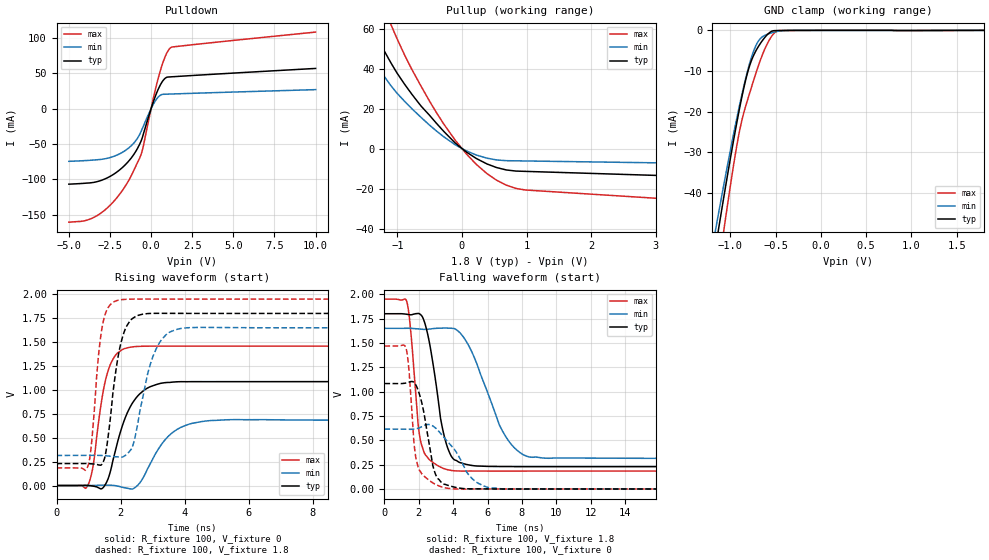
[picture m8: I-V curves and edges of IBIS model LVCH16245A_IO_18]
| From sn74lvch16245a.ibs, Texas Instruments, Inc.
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[Model]   LVCH16245A_IO_18
Model_type  3-state
Enable   Active-Low
Vref =   0
Rref =   1000
Cref =   30p
Vmeas =   0.9
| variable   typ   min   max
C_comp   4.79pF   4.43pF   5.43pF
| C_pullup   5.86pF   3.31pF   12.01pF
| C_pulldown   8.06pF   4.99pF   10.39pF
| C_tri-state   4.79pF   4.43pF   5.43pF
[Temperature Range]   40   100   -40
| Ambient temperature   25   85   -40
[Voltage range]   1.8   1.65   1.95
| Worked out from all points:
|   slope of the pulldown table from 0 to 0.27 V, typ, clamps not added: 14.8 ohm
|   slope of the pullup table from 0 to 0.27 V, typ, clamps not added: 46.5 ohm
|   GND clamp passes 1 mA (typ) near -0.59 V on its own axis
|   rising waveform, R_fixture 100, V_fixture 0: 20-80 % time 652ps typ, 803ps min, 400ps max; typ from 0 V to 1.09 V
|   falling waveform, R_fixture 100, V_fixture 1.8: 20-80 % time 843ps typ, 1.76ns min, 514ps max; typ from 1.8 V to 0.23 V
|   rising waveform, R_fixture 100, V_fixture 1.8: 20-80 % time 385ps typ, 552ps min, 277ps max; typ from 0.229 V to 1.8 V
|   falling waveform, R_fixture 100, V_fixture 0: 20-80 % time 654ps typ, 1.37ns min, 414ps max; typ from 1.08 V to 0 V
[GND Clamp]
| LVCH16245A_IO_18
|   Voltage   I(typ)   I(min)   I(max)
-5V       -657.7mA   -597mA     -758.5mA
-1.165V   -53.4mA    -49.05mA   -63.64mA
-1.13V    -48.59mA   -44.75mA   -58.04mA
-1.065V   -39.83mA   -36.93mA   -47.84mA
-915mV    -20.95mA   -20.02mA   -26.51mA
-860mV    -14.93mA   -14.46mA   -20.87mA
-795mV    -9.18mA    -8.674mA   -15.93mA
-740mV    -5.956mA   -4.853mA   -12.01mA
-675mV    -3.409mA   -2.158mA   -7.673mA
-575mV    -688.2uA   -820.5uA   -2.53mA
-495mV    -55.43uA   -321.6uA   -307.2uA
1.8V      10.89pA    55.22nA    -431pA
[Pulldown]
| LVCH16245A_IO_18
|   Voltage   I(typ)   I(min)   I(max)
-5V       -106.8mA   -74.48mA   -160.5mA
-3.945V   -105.3mA   -73.35mA   -157.9mA
-3.11V    -102mA     -71.9mA    -148.6mA
-2.215V   -91.79mA   -66.95mA   -129.7mA
-1.4V     -75.15mA   -56.3mA    -103.1mA
-920mV    -59.95mA   -44.93mA   -80.72mA
-585mV    -44.32mA   -30.88mA   -63.04mA
60mV      4.341mA    2.845mA    6.529mA
455mV     28.54mA    16.86mA    44.89mA
845mV     42.74mA    20.36mA    72.96mA
1.185V    44.91mA    20.64mA    86.07mA
10V       56.83mA    26.86mA    108.2mA
[Pullup]
| LVCH16245A_IO_18
|   Voltage   I(typ)   I(min)   I(max)
-5V       59.9mA     24.93mA    137.1mA
-3.525V   172.8mA    34.3mA     282.6mA
-3.275V   178.8mA    43.79mA    262.1mA
-3.19V    174.9mA    62.85mA    254.7mA
-1.815V   89.03mA    67.09mA    127mA
-1.63V    76.68mA    57.69mA    108.5mA
-1.365V   58.9mA     44.05mA    84.12mA
-1.1V     43.06mA    31.59mA    62.31mA
-105mV    2.886mA    1.98mA     4.306mA
390mV     -7.662mA   -4.752mA   -12.55mA
835mV     -11.19mA   -6.053mA   -19.89mA
10V       -20.36mA   -10.29mA   -39.14mA
[Ramp]
| LVCH16245A_IO_18
| variable   typ   min   max
dV/dt_r   0.67/6.76E-10   0.44/8.65E-10   0.89/4.15E-10
dV/dt_f   0.94/9.08E-10   0.80/1.91E-09   1.06/5.59E-10
R_load = 100
[Rising Waveform]
| LVCH16245A_IO_18
R_fixture =   100
C_fixture =   0
L_fixture =   0
V_fixture =   0
V_fixture_min = 0
V_fixture_max = 0
|   Time   V(typ)   V(min)   V(max)
0s        -7.691uV   1.503uV    -10.61uV
970ps     1.255mV    -678.4uV   -4.172mV
1.135ns   -5.91mV    493.1uV    187.9mV
1.415ns   -33.15mV   3.634mV    900.4mV
1.635ns   92.92mV    3.696mV    1.224V
2.06ns    628.2mV    -18.62mV   1.422V
2.435ns   893.2mV    -25.6mV    1.452V
3.67ns    1.083V     565mV      1.458V
5.25ns    1.086V     686.7mV    1.458V
49.99ns   1.087V     681.3mV    1.458V
[Falling Waveform]
| LVCH16245A_IO_18
R_fixture =   100
C_fixture =   0
L_fixture =   0
V_fixture =   1.8
V_fixture_min = 1.65
V_fixture_max = 1.95
|   Time   V(typ)   V(min)   V(max)
0s        1.8V       1.65V      1.95V
1.315ns   1.794V     1.651V     1.915V
1.555ns   1.789V     1.65V      1.572V
1.955ns   1.803V     1.645V     673.1mV
2.23ns    1.76V      1.64V      416mV
3.75ns    388.8mV    1.652V     195.1mV
4.935ns   246.2mV    1.462V     184.6mV
7.065ns   230.4mV    536mV      184mV
8.46ns    229.6mV    328mV      184.1mV
49.99ns   229.5mV    314.9mV    184mV
[Rising Waveform]
| LVCH16245A_IO_18
R_fixture =   100
C_fixture =   0
L_fixture =   0
V_fixture =   1.8
V_fixture_min = 1.65
V_fixture_max = 1.95
|   Time   V(typ)   V(min)   V(max)
0s        229.5mV    314.8mV    184mV
1ns       229mV      315.5mV    223.8mV
1.315ns   215.4mV    315.4mV    1.37V
1.445ns   237.7mV    313.5mV    1.691V
2.045ns   1.532V     297.8mV    1.945V
2.365ns   1.745V     396.7mV    1.95V
2.845ns   1.798V     1.165V     1.95V
3.15ns    1.801V     1.454V     1.95V
4.095ns   1.8V       1.65V      1.95V
49.99ns   1.8V       1.65V      1.95V
[Falling Waveform]
| LVCH16245A_IO_18
R_fixture =   100
C_fixture =   0
L_fixture =   0
V_fixture =   0
V_fixture_min = 0
V_fixture_max = 0
|   Time   V(typ)   V(min)   V(max)
0s        1.083V     615mV      1.468V
1.255ns   1.088V     613.8mV    1.447V
1.42ns    1.097V     613.2mV    1.232V
1.805ns   1.075V     617.1mV    347mV
2.21ns    857.1mV    644mV      147.8mV
2.9ns     187.3mV    636.5mV    54.22mV
3.625ns   41.26mV    496.3mV    8.911mV
5.22ns    735uV      87.54mV    403uV
6.95ns    230.3uV    -215.2uV   57.26uV
49.99ns   26.44uV    61.86uV    9.914uV
